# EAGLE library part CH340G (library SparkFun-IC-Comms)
A simple USB 2.0 to Serial IC.
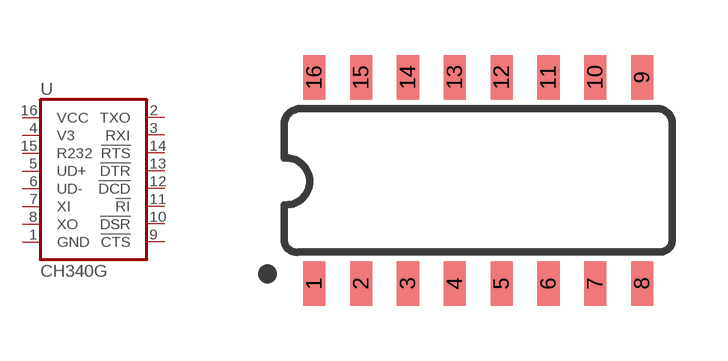
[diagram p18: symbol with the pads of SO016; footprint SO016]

Designator prefix U

## CH340GSMD (PROD_ID: IC-13498; VALUE: CH340G)  [SO016]
1  GND
2  TXO
3  RXI
4  V3
5  UD+
6  UD-
7  XI
8  XO
9  !CTS
10  !DSR
11  !RI
12  !DCD
13  !DTR
14  !RTS
15  R232
16  VCC

## Footprint SO016 (pad centres in mm)
smd 0.6 x 1.2: 1 -4.445,-2.8; 2 -3.175,-2.8; 3 -1.905,-2.8; 4 -0.635,-2.8; 5 0.635,-2.8; 6 1.905,-2.8; 7 3.175,-2.8; 8 4.445,-2.8; 9 4.445,2.8; 10 3.175,2.8; 11 1.905,2.8; 12 0.635,2.8; 13 -0.635,2.8; 14 -1.905,2.8; 15 -3.175,2.8; 16 -4.445,2.8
